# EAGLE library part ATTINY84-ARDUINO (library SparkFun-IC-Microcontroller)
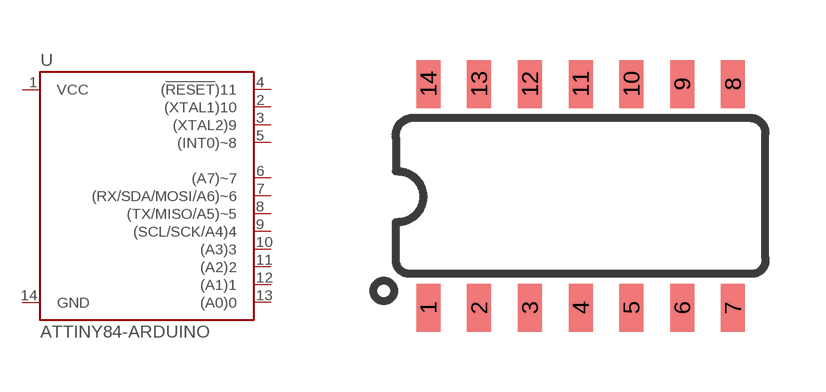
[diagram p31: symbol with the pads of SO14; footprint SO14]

Designator prefix U

## ATTINY84-ARDUINO (PROD_ID: IC-14155)  [SO14]
1  VCC
2  (XTAL1)10
3  (XTAL2)9
4  (!RESET!)11
5  (INT0)~8
6  (A7)~7
7  (RX/SDA/MOSI/A6)~6
8  (TX/MISO/A5)~5
9  (SCL/SCK/A4)4
10  (A3)3
11  (A2)2
12  (A1)1
13  (A0)0
14  GND

## Footprint SO14 (pad centres in mm)
SOIC, 0.15 inch width
smd 0.6 x 1.2: 1 -3.175,-2.8; 2 -1.905,-2.8; 3 -0.635,-2.8; 4 0.635,-2.8; 5 1.905,-2.8; 6 3.175,-2.8; 7 4.445,-2.8; 8 4.445,2.8; 9 3.175,2.8; 10 1.905,2.8; 11 0.635,2.8; 12 -0.635,2.8; 13 -1.905,2.8; 14 -3.175,2.8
